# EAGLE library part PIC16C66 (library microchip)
MICROCONTROLLER
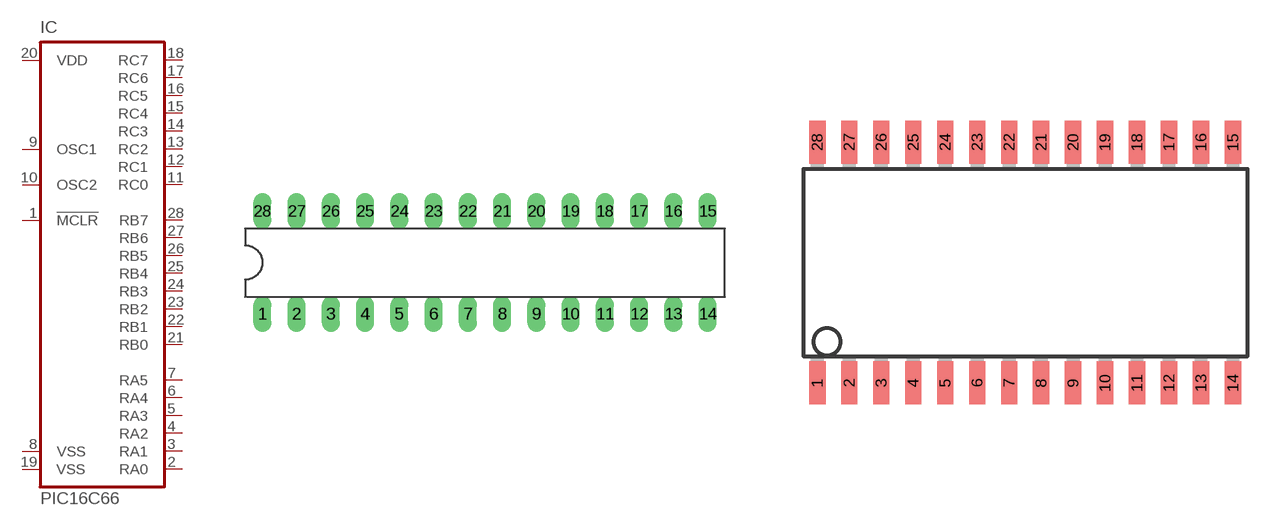
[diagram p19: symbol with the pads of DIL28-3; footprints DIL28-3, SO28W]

Designator prefix IC

## PIC16C66P (MF: MICROCHIP; MPN: PIC16C66-04I/SP; OC_FARNELL: 9759735; OC_NEWARK: 23C4276)  [DIL28-3]
1  !MCLR  in
2  RA0
3  RA1
4  RA2
5  RA3
6  RA4
7  RA5
8  VSS  pwr
9  OSC1
10  OSC2
11  RC0
12  RC1
13  RC2
14  RC3
15  RC4
16  RC5
17  RC6
18  RC7
19  VSS  pwr
20  VDD  pwr
21  RB0
22  RB1
23  RB2
24  RB3
25  RB4
26  RB5
27  RB6
28  RB7

## PIC16C66SO (MPN: PIC16C66-10/SO; OC_FARNELL: 9759727; OC_NEWARK: 97K7254)  [SO28W]
Pads as for DIL28-3

## PIC16C66JW (MF: MICROCHIP; MPN: PIC16C66/JW; OC_FARNELL: 685999; OC_NEWARK: 96K3820)  [DIL28-6]
Pads as for DIL28-3

## Footprint DIL28-3 (pad centres in mm)
Dual In Line package type P
drill 0.813 long: 1 -16.51,-3.81; 2 -13.97,-3.81; 3 -11.43,-3.81; 4 -8.89,-3.81; 5 -6.35,-3.81; 6 -3.81,-3.81; 7 -1.27,-3.81; 8 1.27,-3.81; 9 3.81,-3.81; 10 6.35,-3.81; 11 8.89,-3.81; 12 11.43,-3.81; 13 13.97,-3.81; 14 16.51,-3.81; 15 16.51,3.81; 16 13.97,3.81; 17 11.43,3.81; 18 8.89,3.81; 19 6.35,3.81; 20 3.81,3.81; 21 1.27,3.81; 22 -1.27,3.81; 23 -3.81,3.81; 24 -6.35,3.81; 25 -8.89,3.81; 26 -11.43,3.81; 27 -13.97,3.81; 28 -16.51,3.81

## Footprint SO28W (pad centres in mm)
28-Lead Plastic Small Outline (SO) Wide, 300 mil Body (SOIC) Source: http://ww1.microchip.com/downloads/en/devicedoc/39632c.pdf
smd 0.65 x 1.7: 1 -7.62,-4.78; 2 -6.35,-4.78; 3 -5.08,-4.78; 4 -3.81,-4.78; 5 -2.54,-4.78; 6 -1.27,-4.78; 7 0,-4.78; 8 1.27,-4.78; 9 2.54,-4.78; 10 3.81,-4.78; 11 5.08,-4.78; 12 6.35,-4.78; 13 7.62,-4.78; 14 8.89,-4.78; 15 8.89,4.78; 16 7.62,4.78; 17 6.35,4.78; 18 5.08,4.78; 19 3.81,4.78; 20 2.54,4.78; 21 1.27,4.78; 22 0,4.78; 23 -1.27,4.78; 24 -2.54,4.78; 25 -3.81,4.78; 26 -5.08,4.78; 27 -6.35,4.78; 28 -7.62,4.78

## Footprint DIL28-6 (pad centres in mm)
Dual In Line package type P
drill 0.813 long: 1 -16.51,-7.62; 2 -13.97,-7.62; 3 -11.43,-7.62; 4 -8.89,-7.62; 5 -6.35,-7.62; 6 -3.81,-7.62; 7 -1.27,-7.62; 8 1.27,-7.62; 9 3.81,-7.62; 10 6.35,-7.62; 11 8.89,-7.62; 12 11.43,-7.62; 13 13.97,-7.62; 14 16.51,-7.62; 15 16.51,7.62; 16 13.97,7.62; 17 11.43,7.62; 18 8.89,7.62; 19 6.35,7.62; 20 3.81,7.62; 21 1.27,7.62; 22 -1.27,7.62; 23 -3.81,7.62; 24 -6.35,7.62; 25 -8.89,7.62; 26 -11.43,7.62; 27 -13.97,7.62; 28 -16.51,7.62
